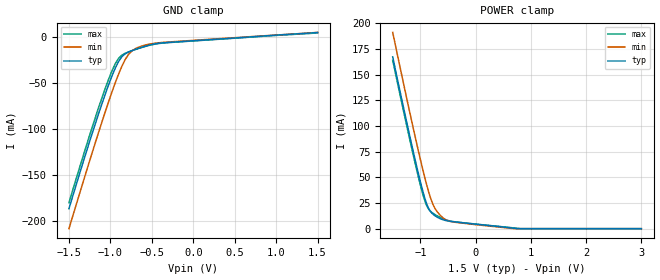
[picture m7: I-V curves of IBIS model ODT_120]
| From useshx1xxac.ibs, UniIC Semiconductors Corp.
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|   Model ODT_120
[Model]  ODT_120
Model_type   Input
Polarity   Non-Inverting
Vinl =   0.600000V
Vinh =   0.900000V
C_comp   1.3900pF   1.3640pF   1.5600pF
[Temperature Range]   25.0000   95.0000   0.0
[Voltage Range]   1.5000V   1.4000V   1.6000V
[GND_clamp]
|Voltage   I(typ)   I(min)   I(max)
-1.5V     -186.6mA   -208.3mA   -180.1mA
-1.18V    -93.98mA   -114.5mA   -87.28mA
-1.06V    -61.93mA   -81.01mA   -55.63mA
-980mV    -42.51mA   -59.81mA   -36.99mA
-940mV    -33.96mA   -49.8mA    -29.25mA
-900mV    -26.79mA   -40.41mA   -23.46mA
-860mV    -21.64mA   -31.9mA    -20mA
-780mV    -16.67mA   -19.19mA   -16.61mA
-740mV    -15.23mA   -15.51mA   -15.32mA
-620mV    -11.55mA   -10.24mA   -11.79mA
-420mV    -7.291mA   -6.758mA   -7.569mA
1.5V      4.361mA    4.536mA    3.926mA
[POWER_clamp]
|Voltage   I(typ)   I(min)   I(max)
-1.5V     167.4mA    191.3mA    164.1mA
-1.12V    73.22mA    95.97mA    69.8mA
-1V       45.94mA    67.67mA    42.67mA
-920mV    29.97mA    49.95mA    27.45mA
-880mV    23.49mA    41.71mA    21.93mA
-840mV    18.68mA    34.14mA    18.39mA
-760mV    13.6mA     22.33mA    14.6mA
-680mV    10.8mA     15.51mA    12.11mA
-580mV    8.517mA    10.14mA    9.587mA
-400mV    6.754mA    6.47mA     6.876mA
752.9mV   0A         NA         NA
3V        0A         0A         0A
